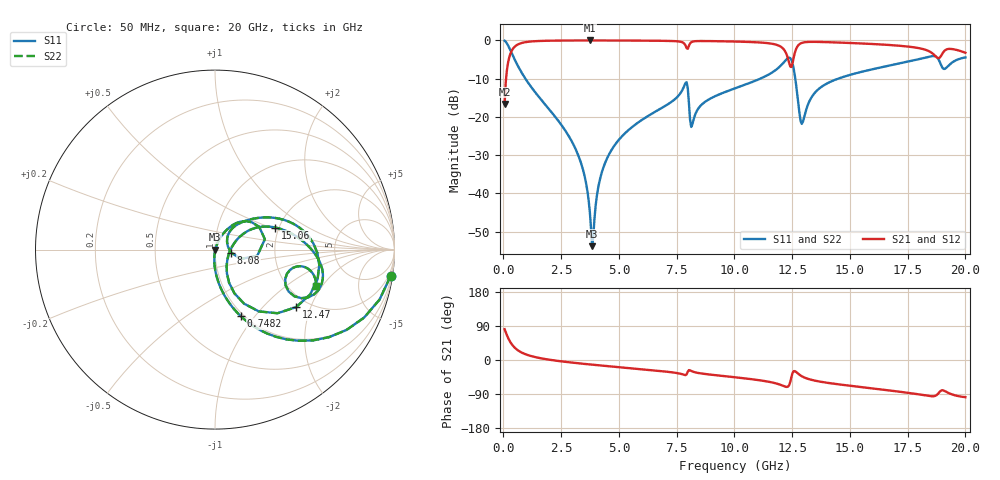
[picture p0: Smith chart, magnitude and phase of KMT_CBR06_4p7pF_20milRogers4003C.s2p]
! Data measured by Modelithics Inc. support@modelithics.com 813-866-6335
! KEMET CBR0603 4.7pF, Pad Width= 0.851mm, Pad Length= 0.64mm, Pad Gap= 0.62mm, 20mil Rogers 4003C substrate Data, January 2022
# hz S ma R 50
! 2 Port Network Data from SP1.SP block
! freq  magS11  angS11  magS21  angS21  magS12  angS12  magS22  angS22
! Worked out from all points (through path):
!   401 points, 50 MHz to 20 GHz, reference 50 ohm
!   highest |S21| = -0.02 dB at 3.741 GHz (marker M1); lowest = -16.6 dB at 50 MHz (marker M2)
!   group delay of S21, straight-line fit = 15.8 ps
!   lowest |S11| = -53.8 dB at 3.841 GHz (marker M3), VSWR 1.00, Z = 50.2 - j0.0906 ohm
!   |S11| at or under -10 dB: 948.3 MHz to 11.12 GHz (10.18 GHz wide, 169 % of centre); 12.63 GHz to 14.5 GHz (1.861 GHz wide, 13.7 % of centre)
!   |S22| runs from -53.8 to -0.1 dB; largest |S21 - S12| = 0
!   S11 on the Smith chart (normalised r, x): 50 MHz: 1, -13; 748.2 MHz: 0.97, -0.85; 8.08 GHz: 1.20, -0.04; 12.47 GHz: 1.72, -1.59; 15.06 GHz: 1.91, +0.54; 20 GHz: 2.77, -1.74
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5e7  0.9891 -8.6  0.1472 81.4  0.1472 81.4  0.9891 -8.6
2.99375e8  0.7442 -42.8  0.6671 47.1  0.6671 47.1  0.7442 -42.8
7.4825e8  0.3968 -68.9  0.9169 21.0  0.9169 21.0  0.3968 -68.9
3.391625e9  0.02311 -95.0  0.9978 -9.6  0.9978 -9.6  0.02311 -95.0
3.74075e9  0.005642 -81.5  0.9979 -11.7  0.9979 -11.7  0.005642 -81.5
3.8405e9  0.002035 -26.3  0.9979 -12.3  0.9979 -12.3  0.002035 -26.3
4.189625e9  0.01574 68.1  0.9977 -14.4  0.9977 -14.4  0.01574 68.1
4.6385e9  0.03517 69.5  0.997 -16.9  0.997 -16.9  0.03517 69.5
6.73325e9  0.1245 59.7  0.9886 -28.7  0.9886 -28.7  0.1245 59.7
7.880375e9  0.2768 27.4  0.86 -40.0  0.86 -40.0  0.2768 27.4
8.079875e9  0.09121 -10.5  0.9121 -27.3  0.9121 -27.3  0.09121 -10.5
1.0025e10  0.236 43.1  0.9659 -45.6  0.9659 -45.6  0.236 43.1
1.192025e10  0.4422 20.5  0.8541 -63.9  0.8541 -63.9  0.4422 20.5
1.246888e10  0.5541 -35.3  0.4488 -44.6  0.4488 -44.6  0.5541 -35.3
1.266838e10  0.2661 -66.1  0.7692 -31.4  0.7692 -31.4  0.2661 -66.1
1.291775e10  0.08083 -17.4  0.926 -42.9  0.926 -42.9  0.08083 -17.4
1.336662e10  0.1858 29.3  0.9572 -52.8  0.9572 -52.8  0.1858 29.3
1.506238e10  0.3581 20.1  0.9235 -68.4  0.9235 -68.4  0.3581 20.1
1.670825e10  0.4683 8.2  0.8707 -80.3  0.8707 -80.3  0.4683 8.2
1.8803e10  0.5837 -27.1  0.5874 -89.9  0.5874 -89.9  0.5837 -27.1
1.930175e10  0.479 -11.1  0.7745 -87.9  0.7745 -87.9  0.479 -11.1
2e10  0.5981 -19.7  0.6886 -98.1  0.6886 -98.1  0.5981 -19.7
